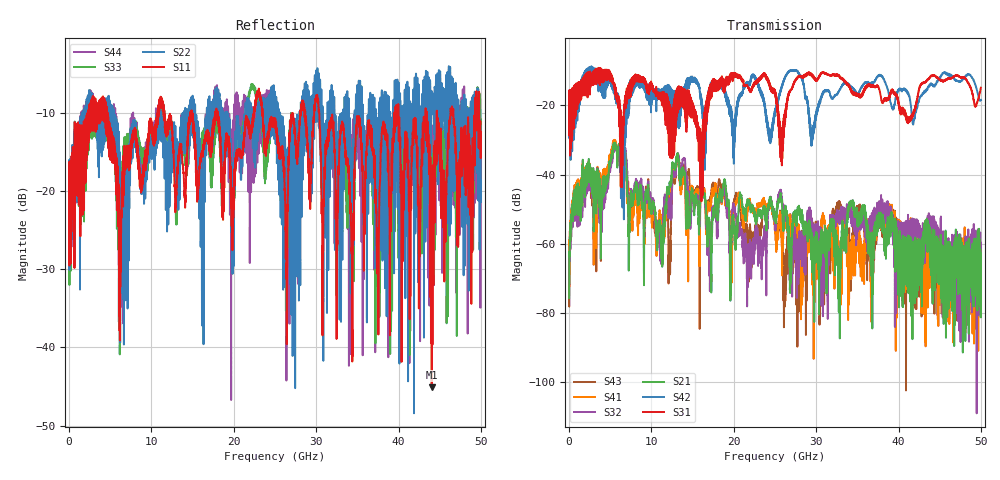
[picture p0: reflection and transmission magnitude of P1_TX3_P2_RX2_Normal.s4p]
!Keysight Technologies,N5225B,MY57041031,A.13.20.10
!Date: Friday, May 31, 2019 11:30:00
!Correction: S11(Full 4 Port(1,2,3,4))
!S12(Full 4 Port(1,2,3,4))
!S13(Full 4 Port(1,2,3,4))
!S14(Full 4 Port(1,2,3,4))
!S21(Full 4 Port(1,2,3,4))
!S22(Full 4 Port(1,2,3,4))
!S23(Full 4 Port(1,2,3,4))
!S24(Full 4 Port(1,2,3,4))
!S31(Full 4 Port(1,2,3,4))
!S32(Full 4 Port(1,2,3,4))
!S33(Full 4 Port(1,2,3,4))
!S34(Full 4 Port(1,2,3,4))
!S41(Full 4 Port(1,2,3,4))
!S42(Full 4 Port(1,2,3,4))
!S43(Full 4 Port(1,2,3,4))
!S44(Full 4 Port(1,2,3,4))
!S4P File: Measurements: <S11,S12,S13,S14>,
!<S21,S22,S23,S24>,
!<S31,S32,S33,S34>,
!<S41,S42,S43,S44>:
# Hz S  dB  R 50.0
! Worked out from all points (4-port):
!   5000 points, 10 MHz to 50 GHz, reference 50 ohm
!   strongest paths, dB at 10 MHz, 12.51 GHz, 25.01 GHz, 37.51 GHz, 50 GHz:
!     S31: -19.4, -27.3, -15.7, -14.5, -14.9
!     S42: -19.4, -16.0, -21.7, -11.5, -18.5
!     S21: -75.6, -38.2, -52.8, -52.5, -65.6
!     S32: -68.4, -43.0, -55.2, -52.6, -64.6
!     S41: -59.0, -39.0, -55.3, -51.7, -62.7
!     S43: -71.8, -44.2, -53.9, -52.4, -64.6
!   lowest |S11| = -45.1 dB at 44.03 GHz (marker M1), VSWR 1.01, Z = 49.8 + j0.501 ohm
!   |S11| at or under -10 dB: 4.66 GHz to 10.77 GHz (6.106 GHz wide, 79.2 % of centre); 23.49 GHz to 28.08 GHz (4.582 GHz wide, 17.8 % of centre); 30.37 GHz to 39.5 GHz (9.122 GHz wide, 26.1 % of centre)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
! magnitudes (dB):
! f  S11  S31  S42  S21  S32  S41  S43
! 10 MHz  -19.6  -19.4  -19.4  -75.6  -68.4  -59.0  -71.8
! 5.56 GHz  -16.0  -14.1  -15.7  -31.5  -32.4  -30.6  -31.7
! 11.17 GHz  -8.2  -17.3  -17.2  -60.3  -63.4  -54.9  -59.7
! 13.2 GHz  -17.1  -15.2  -18.1  -33.9  -33.8  -34.2  -33.8
! 21.85 GHz  -11.4  -15.3  -14.2  -48.0  -62.2  -48.0  -62.8
! 44.03 GHz  -45.1  -11.4  -14.1  -63.1  -57.5  -59.5  -59.5
! 50 GHz  -12.5  -14.9  -18.5  -65.6  -64.6  -62.7  -64.6
